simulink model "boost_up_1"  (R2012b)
settings: Solver=ode45  StartTime=0.0  StopTime=10.0  RelTol=1e-3
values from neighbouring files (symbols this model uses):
  C = 100e-6    (= 0.0001)    [boost_up1.m]    (also in buck_boost1.m = 0.0002; buck_boost2.m = 0.0002; buck_down1.m; buck_down2.m)
  f0 = 0.2e5    (= 20000)    [boost_up1.m]    (also in buck_boost1.m; buck_boost2.m; buck_down1.m; buck_down2.m)
  L = 0.001    [boost_up1.m]    (also in buck_boost1.m; buck_boost2.m; buck_down1.m; buck_down2.m)
  R = 5    [boost_up1.m]    (also in buck_boost1.m; buck_boost2.m; buck_down1.m = 2*Rmax,; buck_down2.m = 0.1*Rmax,)
  Ui = 5    [boost_up1.m]    (also in buck_boost1.m; buck_boost2.m; buck_down1.m; buck_down2.m)

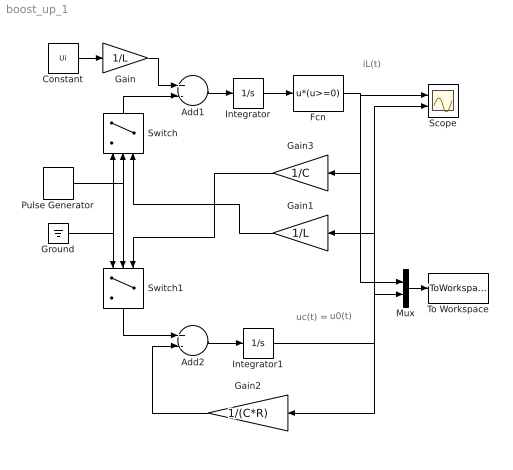
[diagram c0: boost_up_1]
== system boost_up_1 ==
  note: uc(t) =
  note: iL(t)
  note: u0(t)
  Add1 : Sum  Inputs=+-
  Add2 : Sum  Inputs=+-
  Constant : Constant  Value=Ui
  Fcn : Fcn  Expr=u*(u>=0)
  Gain : Gain  Gain=1/L
  Gain1 : Gain  Gain=1/L
  Gain2 : Gain  Gain=1/(C*R)
  Gain3 : Gain  Gain=1/C
  Ground : Ground
  Integrator : Integrator
  Integrator1 : Integrator
  Mux : Mux  Inputs=2
  Pulse Generator : DiscretePulseGenerator  PulseType=Time based  Period=1/f0  PulseWidth=50
  Scope : Scope  NumInputPorts=2
  Switch : Switch  Criteria=u2 > Threshold  Threshold=0.5  ZeroCross=off  SampleTime=0
  Switch1 : Switch  Criteria=u2 > Threshold  Threshold=0.5  ZeroCross=off  SampleTime=0
  To Workspace : ToWorkspace  VariableName=y  SampleTime=-1  SaveFormat=Structure With Time
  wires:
  Ground/1 -> Switch1/1, Switch/1
  Pulse Generator/1 -> Switch1/2, Switch/2
  Switch/1 -> Add1/2
  Constant/1 -> Gain/1
  Gain/1 -> Add1/1
  Switch1/1 -> Add2/1
  Add1/1 -> Integrator/1
  Integrator/1 -> Fcn/1
  Fcn/1 -> Scope/1, Mux/1, Gain3/1
  Gain3/1 -> Switch1/3
  Add2/1 -> Integrator1/1
  Gain1/1 -> Switch/3
  Gain2/1 -> Add2/2
  Integrator1/1 -> Gain2/1, Mux/2, Scope/2, Gain1/1
  Mux/1 -> To Workspace/1
